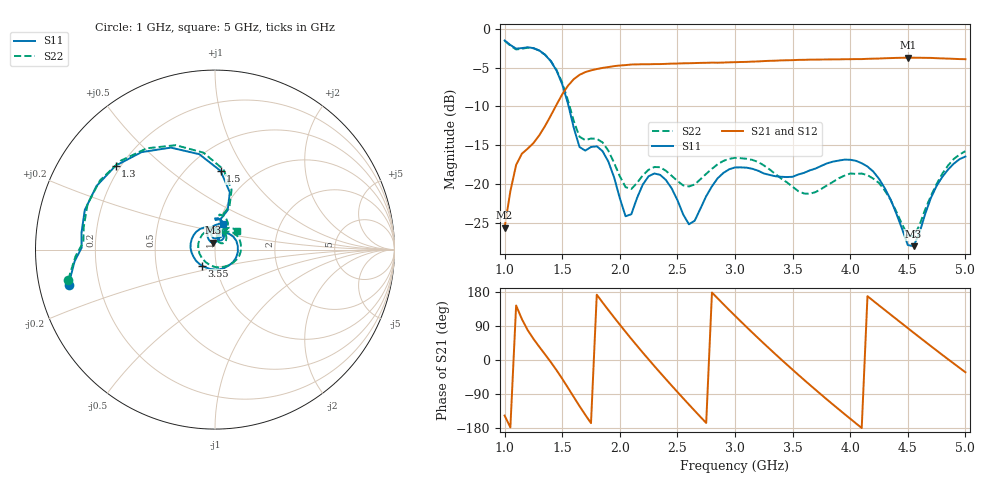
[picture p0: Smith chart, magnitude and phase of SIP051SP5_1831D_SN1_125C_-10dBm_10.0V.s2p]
# GHz  S  dB  R  50
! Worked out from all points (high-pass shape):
!   81 points, 1 GHz to 5 GHz, reference 50 ohm
!   highest |S21| = -3.74 dB at 4.5 GHz (marker M1); lowest = -25.6 dB at 1 GHz (marker M2)
!   |S21| within 3 dB of the highest: 1.586 GHz to end of sweep
!   lowest |S11| = -27.9 dB at 4.55 GHz (marker M3), VSWR 1.08, Z = 48.8 + j3.77 ohm
!   |S11| at or under -10 dB: 1.556 GHz to end of sweep
!   |S22| runs from -26.7 to -1.6 dB; largest |S21 - S12| = 0.0024
!   S11 on the Smith chart (normalised r, x): 1 GHz: 0.09, -0.12; 1.3 GHz: 0.18, +0.36; 1.5 GHz: 0.71, +0.78; 3.55 GHz: 0.85, -0.16; 5 GHz: 1.05, +0.31
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1  -1.52 -166.5  -25.56 -146.6  -25.52 -146.9  -1.56 -168.4
1.1  -2.58 179.2  -17.51 143.9  -17.49 144.0  -2.68 176.7
1.3  -2.80 139.8  -13.72 35.2  -13.71 35.3  -2.83 136.7
1.5  -7.13 85.9  -8.45 -49.4  -8.44 -49.4  -6.95 84.0
1.6  -12.72 72.1  -6.50 -97.5  -6.48 -97.5  -11.86 71.6
1.7  -15.66 88.7  -5.59 -144.5  -5.58 -144.6  -14.31 83.1
1.85  -15.73 76.0  -5.05 151.9  -5.06 151.9  -14.61 70.8
2  -21.77 62.7  -4.74 93.4  -4.73 93.4  -18.96 60.5
2.2  -20.01 101.4  -4.58 19.3  -4.57 19.4  -18.83 81.1
2.35  -18.78 74.8  -4.56 -33.3  -4.53 -33.4  -17.79 65.4
2.55  -23.85 54.5  -4.46 -101.0  -4.45 -101.0  -20.12 53.6
2.75  -21.51 76.0  -4.39 -166.1  -4.39 -166.1  -18.65 56.9
3  -17.83 22.1  -4.31 116.7  -4.31 116.7  -16.59 22.9
3.3  -18.78 -62.9  -4.14 29.6  -4.14 29.6  -18.08 -35.7
3.55  -18.73 -128.6  -4.02 -39.2  -4.02 -39.1  -20.87 -107.4
3.7  -17.96 -162.2  -3.98 -78.8  -3.98 -78.8  -20.98 -164.8
4.05  -16.97 125.5  -3.92 -167.2  -3.92 -167.2  -18.65 92.6
4.35  -21.92 73.4  -3.79 120.1  -3.79 120.1  -21.97 40.1
4.5  -27.79 85.4  -3.74 84.1  -3.74 84.2  -26.51 49.2
4.55  -27.93 105.7  -3.74 72.2  -3.74 72.2  -26.66 64.2
4.8  -19.03 108.3  -3.83 13.4  -3.83 13.5  -18.61 70.5
5  -16.43 71.9  -3.93 -32.3  -3.93 -32.3  -15.73 40.4
